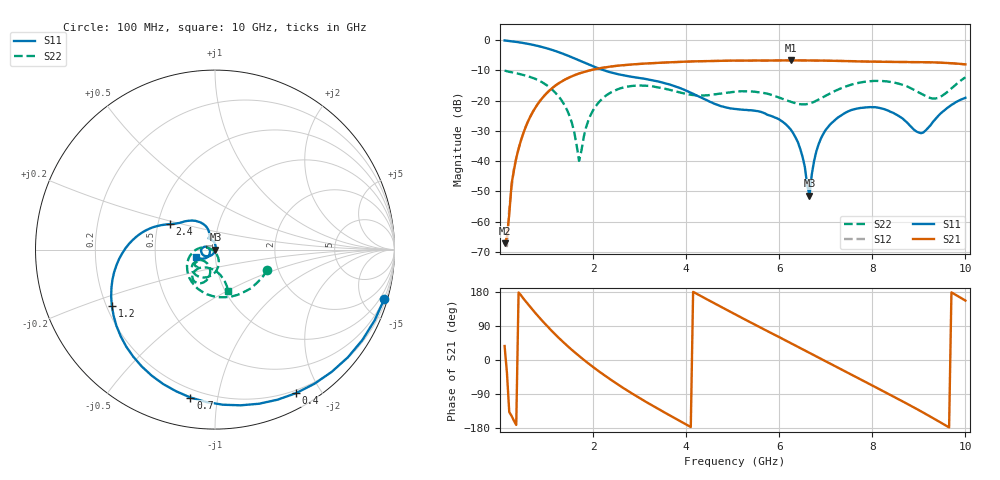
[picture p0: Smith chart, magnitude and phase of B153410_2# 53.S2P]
!  2-Port S-parameters saved by WinCal
! VAR MeasName=S-Parameters (CALIBRATED_DATA) read from VNA (N5245A)
! VAR MeasDate=2016-12-23 10:02:10
! VAR NAME=B153410_2# 53
! VAR FILENAME=B153410_2# 53.S2P
! VAR DATE=2016-12-23 10:02:10
! VAR PHYS_PORTS=1,2
# Hz S DB R 50
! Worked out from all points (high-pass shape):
!   199 points, 100 MHz to 10 GHz, reference 50 ohm
!   highest |S21| = -6.72 dB at 6.25 GHz (marker M1); lowest = -67.1 dB at 100 MHz (marker M2)
!   |S21| within 3 dB of the highest: 2.016 GHz to end of sweep
!   lowest |S11| = -51.4 dB at 6.65 GHz (marker M3), VSWR 1.01, Z = 50.2 - j0.121 ohm
!   |S11| at or under -10 dB: 2.234 GHz to end of sweep
!   |S22| runs from -39.9 to -10.1 dB; largest |S21 - S12| = 0.0018
!   S11 on the Smith chart (normalised r, x): 100 MHz: 0.44, -7.01; 400 MHz: 0.17, -1.70; 700 MHz: 0.15, -0.84; 1.2 GHz: 0.22, -0.24; 2.4 GHz: 0.58, +0.18; 10 GHz: 0.81, -0.06
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1e8  -0.15 -16.2  -67.13 37.0  -66.25 44.4  -10.08 -21.2
1.5e8  -0.24 -23.9  -65.00 -33.7  -68.06 -61.1  -10.29 -30.3
3e8  -0.52 -46.3  -43.05 -160.2  -42.32 -166.3  -10.86 -55.4
4e8  -0.74 -60.5  -35.94 178.2  -35.76 179.1  -11.15 -71.2
7e8  -1.56 -99.4  -23.91 132.9  -23.86 132.9  -12.45 -113.6
1.2e9  -3.68 -151.3  -14.95 66.0  -14.91 66.1  -17.56 -170.1
1.5e9  -5.42 -174.6  -12.29 31.6  -12.25 31.5  -25.27 167.1
1.7e9  -6.71 173.4  -11.05 10.7  -11.05 10.5  -39.88 -140.8
1.75e9  -7.04 170.8  -10.82 5.6  -10.80 5.4  -36.52 -89.4
1.95e9  -8.34 162.2  -9.95 -13.8  -9.95 -13.9  -24.68 -69.9
2.4e9  -10.76 150.6  -8.71 -53.6  -8.72 -53.7  -17.19 -95.1
3.4e9  -13.69 128.4  -7.55 -129.0  -7.55 -129.1  -15.61 -141.1
5.05e9  -22.77 118.6  -6.81 120.7  -6.83 120.8  -17.07 -137.9
6.25e9  -29.60 90.1  -6.72 44.4  -6.74 44.4  -20.39 -142.0
6.5e9  -38.47 70.4  -6.73 28.3  -6.74 28.4  -21.23 -127.2
6.65e9  -51.44 -26.7  -6.76 18.7  -6.75 18.8  -20.99 -117.5
6.7e9  -44.37 -82.5  -6.75 15.5  -6.76 15.5  -20.70 -114.4
6.9e9  -32.38 -112.7  -6.79 2.6  -6.80 2.7  -19.23 -105.0
7.25e9  -25.71 -133.8  -6.90 -19.7  -6.89 -19.7  -16.46 -102.0
8.35e9  -23.37 169.9  -7.24 -89.6  -7.24 -89.5  -13.74 -126.7
9.05e9  -30.77 -166.7  -7.31 -135.7  -7.31 -135.7  -17.73 -128.7
1e10  -19.08 -159.6  -8.04 156.9  -8.05 156.9  -12.31 -72.3
